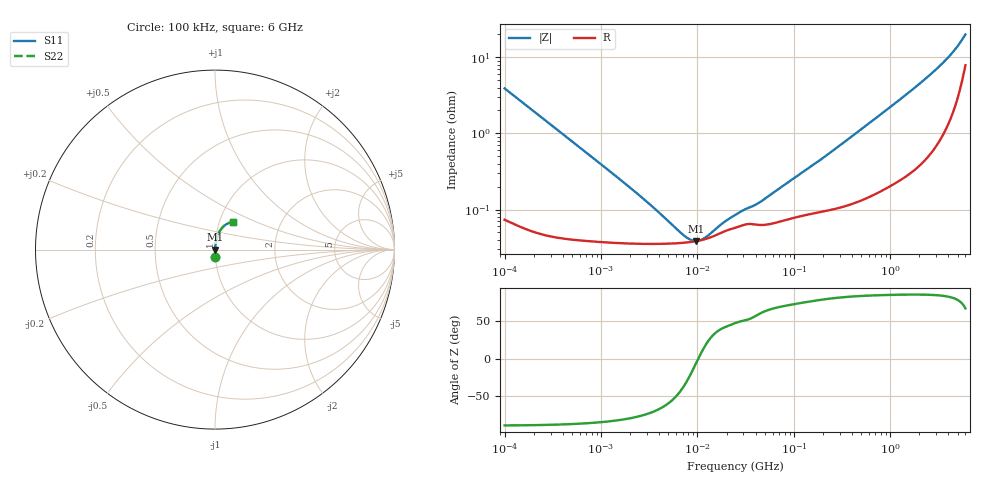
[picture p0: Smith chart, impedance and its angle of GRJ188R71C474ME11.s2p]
!Murata Part Number: GRJ188R71C474ME11
!These Parameters are Measured in Series Mode Connection
!Data Generated on Jun 19, 2026
!  o--ll--o
!Port1  Port2
!  o------o
!Operation Temp=25[degC], DC Bias Voltage=0[V]
!Freq. Start=100[kHz] Stop=6[GHz] 401[Steps]
# Hz S RI R 50
!Freq.(Hz) S11(Real) S11(Imag) S21(Real) S21(Imag) S12(Real) S12(Imag) S22(Real) S22(Imag)
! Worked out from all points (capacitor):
!   401 points, 100 kHz to 6 GHz, reference 50 ohm
!   read as one part in series: C = 407 nF near 105.7 kHz
!   lowest |Z| = 38.6 mohm at 9.615 MHz (marker M1)
!   series resonance near 10.2 MHz, so ESL is about 600 pH
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100000  0.00225 -0.0389  0.9978 0.0389  0.9978 0.0389  0.00225 -0.0389
105655  0.00207 -0.0368  0.9979 0.0368  0.9979 0.0368  0.00207 -0.0368
631452  0.000429 -0.00621  0.9996 0.00621  0.9996 0.00621  0.000429 -0.00621
2004685  0.00036 -0.0019  0.9996 0.0019  0.9996 0.0019  0.00036 -0.0019
3987316  0.000354 -0.000842  0.9996 0.000842  0.9996 0.000842  0.000354 -0.000842
7302625  0.000366 -0.000264  0.9996 0.000264  0.9996 0.000264  0.000366 -0.000264
8379264  0.000373 -0.000153  0.9996 0.000153  0.9996 0.000153  0.000373 -0.000153
9614634  0.000383 -4.54e-05  0.9996 4.54e-05  0.9996 4.54e-05  0.000383 -4.54e-05
1.073283e7  0.000394 3.94e-05  0.9996 -3.94e-05  0.9996 -3.94e-05  0.000394 3.94e-05
1.198108e7  0.000408 0.000124  0.9996 -0.000124  0.9996 -0.000124  0.000408 0.000124
1.860466e7  0.000509 0.000442  0.9995 -0.000442  0.9995 -0.000442  0.000509 0.000442
2.517799e7  0.000581 0.000638  0.9994 -0.000638  0.9994 -0.000638  0.000581 0.000638
4.36444e7  0.000628 0.00106  0.9994 -0.00106  0.9994 -0.00106  0.000628 0.00106
1.546735e8  0.000893 0.00366  0.9991 -0.00366  0.9991 -0.00366  0.000893 0.00366
2.992988e8  0.0011 0.00685  0.9989 -0.00685  0.9989 -0.00685  0.0011 0.00685
9.76689e8  0.00246 0.0216  0.9975 -0.0216  0.9975 -0.0216  0.00246 0.0216
1.889928e9  0.00525 0.0416  0.9948 -0.0416  0.9948 -0.0416  0.00525 0.0416
3.016594e9  0.0117 0.0687  0.9883 -0.0687  0.9883 -0.0687  0.0117 0.0687
3.863894e9  0.0206 0.0919  0.9794 -0.0919  0.9794 -0.0919  0.0206 0.0919
4.68428e9  0.0363 0.1174  0.9637 -0.1174  0.9637 -0.1174  0.0363 0.1174
5.678851e9  0.0769 0.1483  0.9231 -0.1483  0.9231 -0.1483  0.0769 0.1483
6e9  0.0988 0.1532  0.9012 -0.1532  0.9012 -0.1532  0.0988 0.1532
